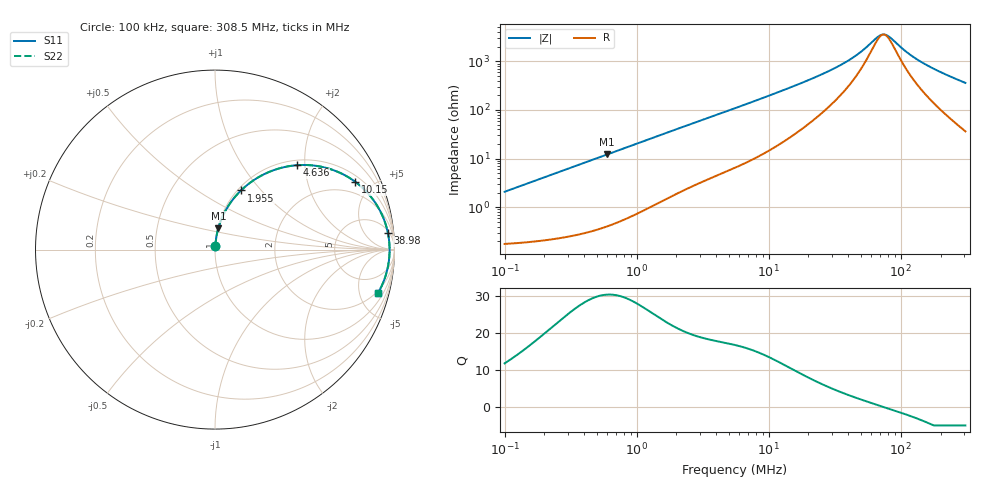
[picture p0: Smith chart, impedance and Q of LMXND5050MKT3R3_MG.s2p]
! LMXND5050MKT3R3_MG  S-PARAMETER MODEL  ( General Type )
! Model Generated by TAIYO YUDEN Corporation (https://www.yuden.co.jp/en/)
! Version 1.0
! TAIYO YUDEN Control No. 191023NI43SB-FBB
! Copyright(c) 2019 TAIYO YUDEN CO.,LTD. All Rights Reserved.
! Product Description (link to TY-COMPAS)
! https://ds.yuden.co.jp/TYCOMPAS/or/detail?pn=LMXND5050MKT3R3MMG&u=M
! Products Name : Inductors
! Characteristics :
!  Inductance : 3.3 uH , SRF(min) : 48 MHz , DC Resistance(max) : 0.192 Ohm
!  Rated Current : Saturation :2400 mA , Temp Rise : 1450 mA (40 degC)
!  Case Size : 4.9 x 4.9 / 0.193 x 0.193 [mm/inch] , Thickness : 1.2 / 0.047 [mm/inch]
!  (Conditions: Temperature = 25 degC , DC Bias Current/Voltage = 0A / 0V)
! External Node Assignments :
!  1  o---GGG---o  2
! GND o---------o GND
! Frequency Range : 0.1MHz  -  308.54851MHz  [ 402 STEP ]
# MHz S RI R 50
! Freq[MHz].  S11 Real  S11 Imag  S21 Real  S21 Imag  S12 Real  S12 Imag  S22 Real  S22 Imag
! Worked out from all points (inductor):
!   401 points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, 100 kHz to 308.5 MHz, reference 50 ohm
!   read as one part in series: L = 3.29 uH near 104.1 kHz
!   highest Q = 30.4 at 597.5 kHz (marker M1), where L = 3.26 uH
!   self-resonance near 74.11 MHz
!   S11 on the Smith chart (normalised r, x): 100 kHz: 1.00, +0.04; 1.955 MHz: 1.04, +0.78; 4.636 MHz: 1.10, +1.82; 10.15 MHz: 1.30, +3.97; 38.98 MHz: 7, +19; 308.5 MHz: 1.73, -7.18
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0.1  0.00218 0.0206  0.9978 -0.0206  0.9978 -0.0206  0.00218 0.0206
0.384115  0.00894 0.0779  0.9911 -0.0779  0.9911 -0.0779  0.00894 0.0779
0.59755  0.0186 0.1195  0.9814 -0.1195  0.9814 -0.1195  0.0186 0.1195
0.987318  0.0451 0.1906  0.9549 -0.1906  0.9549 -0.1906  0.0451 0.1906
1.475446  0.0911 0.2678  0.9089 -0.2678  0.9089 -0.2678  0.0911 0.2678
1.954563  0.1449 0.3296  0.8551 -0.3296  0.8551 -0.3296  0.1449 0.3296
2.920894  0.2627 0.4146  0.7373 -0.4146  0.7373 -0.4146  0.2627 0.4146
4.636091  0.4553 0.4701  0.5447 -0.4701  0.5447 -0.4701  0.4553 0.4701
5.667415  0.5483 0.4686  0.4517 -0.4686  0.4517 -0.4686  0.5483 0.4686
10.14754  0.7816 0.3776  0.2184 -0.3776  0.2184 -0.3776  0.7816 0.3776
14.27767  0.8683 0.2946  0.1317 -0.2946  0.1317 -0.2946  0.8683 0.2946
21.33651  0.9271 0.2013  0.0729 -0.2013  0.0729 -0.2013  0.9271 0.2013
30.02062  0.9529 0.1343  0.0471 -0.1343  0.0471 -0.1343  0.9529 0.1343
38.97828  0.9638 0.0906  0.0362 -0.0906  0.0362 -0.0906  0.9638 0.0906
49.60236  0.9695 0.0547  0.0305 -0.0547  0.0305 -0.0547  0.9695 0.0547
68.40302  0.9726 0.0107  0.0274 -0.0107  0.0274 -0.0107  0.9726 0.0107
74.12565  0.9728 -2.48e-05  0.0272 2.48e-05  0.0272 2.48e-05  0.9728 -2.48e-05
81.95682  0.9726 -0.0134  0.0274 0.0134  0.0274 0.0134  0.9726 -0.0134
110.7732  0.9698 -0.0548  0.0302 0.0548  0.0302 0.0548  0.9698 -0.0548
140.966  0.9644 -0.0908  0.0356 0.0908  0.0356 0.0908  0.9644 -0.0908
202.3643  0.9481 -0.1533  0.0519 0.1533  0.0519 0.1533  0.9481 -0.1533
308.5485  0.9075 -0.2435  0.0925 0.2435  0.0925 0.2435  0.9075 -0.2435
